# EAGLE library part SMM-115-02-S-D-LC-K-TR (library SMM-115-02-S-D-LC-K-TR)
Headers & Wire Housings Low Profile Socket Strips, 2.00 mm Pitch Source: Datasheet
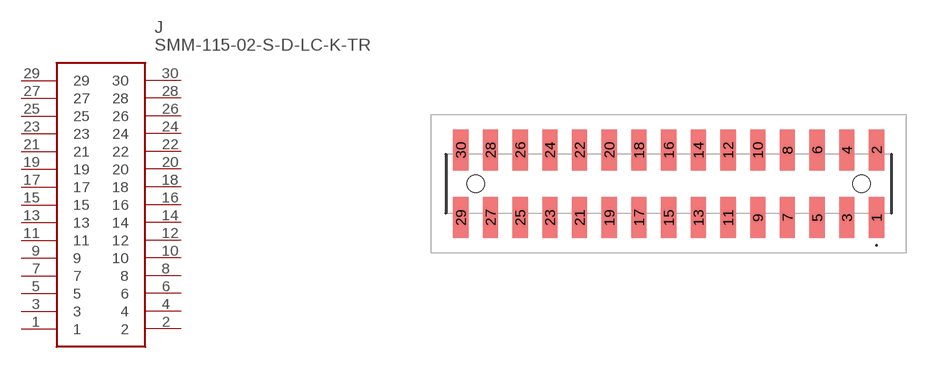
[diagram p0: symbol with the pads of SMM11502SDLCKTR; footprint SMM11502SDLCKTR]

Designator prefix J

## SMM-115-02-S-D-LC-K-TR (Description: Headers & Wire Housings Low Profile Socket Strips, 2.00 mm Pitch; Height: 3.81mm; Manufacturer_Name: SAMTEC; Manufacturer_Part_Number: SMM-115-02-S-D-LC-K-TR; Mouser_Part_Number: 200-SMM11502SDLCKTR; Mouser_Price-Stock: https://www.mouser.co.uk/ProductDetail/Samtec/SMM-115-02-S-D-LC-K-TR?qs=Cqqh%252BS766wmCL5XLNTE7Jg%3D%3D)  [SMM11502SDLCKTR]
1  1
2  2
3  3
4  4
5  5
6  6
7  7
8  8
9  9
10  10
11  11
12  12
13  13
14  14
15  15
16  16
17  17
18  18
19  19
20  20
21  21
22  22
23  23
24  24
25  25
26  26
27  27
28  28
29  29
30  30

## Footprint SMM11502SDLCKTR (pad centres in mm)
SMM-115-02-S-D-LC-K-TR-2
smd 1.02 x 2.77: 1 14,-2.275; 2 14,2.275; 3 12,-2.275; 4 12,2.275; 5 10,-2.275; 6 10,2.275; 7 8,-2.275; 8 8,2.275; 9 6,-2.275; 10 6,2.275; 11 4,-2.275; 12 4,2.275; 13 2,-2.275; 14 2,2.275; 15 0,-2.275; 16 0,2.275; 17 -2,-2.275; 18 -2,2.275; 19 -4,-2.275; 20 -4,2.275; 21 -6,-2.275; 22 -6,2.275; 23 -8,-2.275; 24 -8,2.275; 25 -10,-2.275; 26 -10,2.275; 27 -12,-2.275; 28 -12,2.275; 29 -14,-2.275; 30 -14,2.275
hole 1.19 at 13,0
hole 1.19 at -13,0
